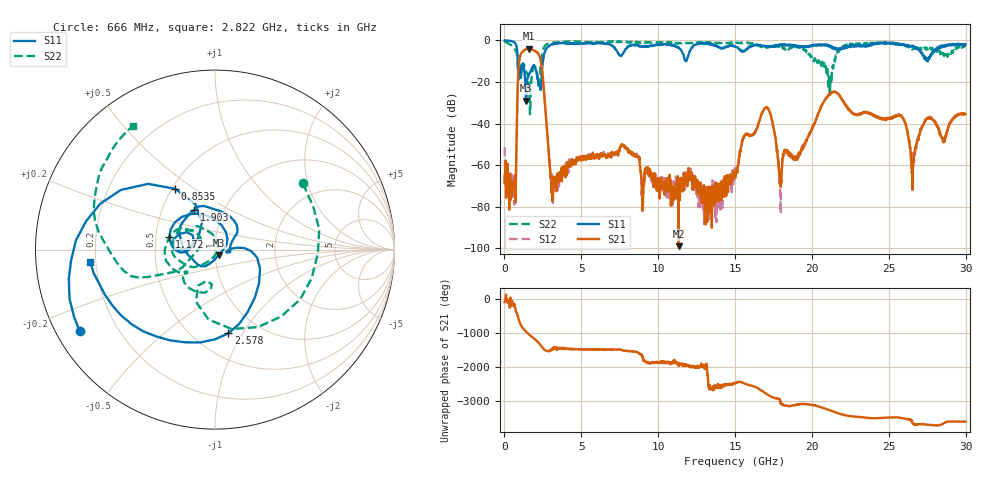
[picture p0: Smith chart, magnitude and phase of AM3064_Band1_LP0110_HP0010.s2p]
# Hz S DB R 50.0
!freq dBS11 angS11 dBS21 angS21 dBS12 angS12 dBS22 angS22
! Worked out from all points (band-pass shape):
!   1600 points, 10 MHz to 29.98 GHz, reference 50 ohm
!   highest |S21| = -4.02 dB at 1.584 GHz (marker M1); lowest = -98.9 dB at 11.33 GHz (marker M2)
!   |S21| within 3 dB of the highest: 1.043 GHz to 2.247 GHz (1.203 GHz wide, 73.2 % of centre)
!   lowest |S11| = -29.0 dB at 1.416 GHz (marker M3), VSWR 1.07, Z = 52 - j3.04 ohm
!   |S11| at or under -10 dB: 865.6 MHz to 2.507 GHz (1.642 GHz wide, 97.3 % of centre); 11.81362 GHz to 11.82084 GHz (7.225 MHz wide, 0.0611 % of centre); 27.52352 GHz to 27.53501 GHz (11.48 MHz wide, 0.0417 % of centre)
!   |S22| runs from -35.5 to -0.4 dB; largest |S21 - S12| = 0.0087
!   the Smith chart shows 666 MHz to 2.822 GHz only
!   S11 on the Smith chart (normalised r, x): 666 MHz: 0.07, -0.28; 853.5 MHz: 0.52, +0.42; 1.172 GHz: 0.59, +0.09; 1.903 GHz: 0.72, +0.34; 2.578 GHz: 0.72, -0.87; 2.822 GHz: 0.18, -0.05
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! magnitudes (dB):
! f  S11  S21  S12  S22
! 10 MHz  0.0  -65.1  -51.4  -0.4
! 666 MHz  -1.1  -69.6  -71.1  -4.3
! 853.5 MHz  -7.8  -24.7  -24.5  -10.2
! 1.172 GHz  -11.6  -5.5  -5.4  -11.5
! 1.416 GHz  -29.0  -4.2  -4.1  -15.7
! 1.584 GHz  -16.4  -4.0  -4.0  -20.8
! 1.903 GHz  -12.0  -4.8  -4.8  -12.4
! 2.578 GHz  -6.5  -25.1  -25.1  -3.2
! 2.822 GHz  -3.1  -47.7  -47.9  -1.7
! 3.271 GHz  -1.5  -68.3  -67.3  -0.9
! 5.015 GHz  -1.4  -55.7  -55.5  -0.6
! 10 GHz  -2.0  -68.2  -67.5  -1.0
! 11.33 GHz  -3.4  -98.9  -68.6  -1.2
! 15 GHz  -2.9  -65.0  -66.4  -1.4
! 16.97 GHz  -2.8  -32.4  -32.4  -3.1
! 17.93 GHz  -2.1  -67.1  -70.4  -2.8
! 19.99 GHz  -2.9  -42.8  -42.7  -8.4
! 21.43 GHz  -4.2  -24.7  -24.6  -9.4
! 25 GHz  -1.0  -37.8  -37.6  -1.2
! 26.57 GHz  -2.6  -60.9  -58.2  -3.9
! 27.49 GHz  -8.7  -37.5  -37.4  -4.0
! 29.98 GHz  -1.9  -35.4  -35.6  -2.9
